DATA_BLOCK DB 15
TITLE =BLOCK DATA FOR TIMER
AUTHOR : Esposito
FAMILY : EGAL_srl
NAME : DB_TD_OP
VERSION : 0.1


  STRUCT
   Axis_press : INT ;	//Value degrees axis rotary press
   Count_tot_R : DINT ;	//Value counter totaly press - read
   Count_par_R : DINT ;	//Value counter partial press - read
   Count_mainte_R : DINT ;	//Value counter maintenance press - read
   Count_par_W : DINT ;	//Value counter partial press - write
   Count_totaly_W : DINT ;	//Value counter totaly - write
   Cam_zero_ON : INT ;	//Value start cam zero - write
   Cam_zero_OFF : INT ;	//Value stop cam zero - write
   Cam_one_ON : INT ;	//Value start cam one - write
   Cam_one_OFF : INT ;	//Value stop cam one - write
   Cam_two_ON : INT ;	//Value start cam two - write
   Cam_two_OFF : INT ;	//Value stop cam two - write
   Cam_three_ON : INT ;	//Value start cam three - write
   Cam_three_OFF : INT ;	//Value stop cam three - write
   Cam_four_ON : INT ;	//Value start cam four - write
   Cam_four_OFF : INT ;	//Value stop cam four - write
   Cam_five_ON : INT ;	//Value start cam five - write
   Cam_five_OFF : INT ;	//Value stop cam five - write
   Cam_six_ON : INT ;	//Value start cam six - write
   Cam_six_OFF : INT ;	//Value stop cam six - write
   Cam_seven_ON : INT ;	//Value start cam seven - write
   Cam_seven_OFF : INT ;	//Value stop cam seven - write
   Cam_eight_ON : INT ;	//Value start cam eight - write
   Cam_eight_OFF : INT ;	//Value stop cam eight - write
   Cam_nine_ON : INT ;	//Value start cam nine - write
   Cam_nine_OFF : INT ;	//Value stop cam nine - write
   Cam_ten_ON : INT ;	//Value start cam ten - write
   Cam_ten_OFF : INT ;	//Value stop cam ten - write
   Cam_eleven_ON : INT ;	//Value start cam eleven - write
   Cam_eleven_OFF : INT ;	//Value stop cam eleven - write
   Cam_twelve_ON : INT ;	//Value start cam twelve - write
   Cam_twelve_OFF : INT ;	//Value stop cam twelve - write
   Cam_thirteen_ON : INT ;	//Value start cam thirteen - write
   Cam_thirteen_OFF : INT ;	//Value stop cam thirteen - write
   Lub_time_pause_R : INT ;	//Value time pause, lubrication pump trabon balancing - read
   Lub_time_job_R : INT ;	//Value time job, lubrication pump trabon balancing - read
   Lub_time_pause_W : INT ;	//Value time pause, lubrication pump trabon balancing - write
   Lub_time_job_W : INT ;	//Value time job, lubrication pump trabon balancing - write
   Overload_POINT1 : REAL ;	//Value point one, pressure overload slide
   Overload_POINT2 : REAL ;	//Value point two, pressure overload slide
   Overload_POINT3 : REAL ;	//Value point three, pressure overload slide
   Overload_POINT4 : REAL ;	//Value point four, pressure overload slide
   Overload_PIW296_R : REAL ;	//Value air pressure, pilotage overload
   Overload_TON288_R : REAL ;	//Value tons overload point one - read
   Overload_TON290_R : REAL ;	//Value tons overload point two - read
   Overload_TON292_R : REAL ;	//Value tons overload point three - read
   Overload_TON294_R : REAL ;	//Value tons overload point four - read
   Ovload_TON_totaly : REAL ;	//Value tons overload totaly slide press - read
   Overload_valve_W : REAL ;	//Value set proportional valve, overload adjustment - write
   Balancing_PIW298_R : REAL ;	//Value air pressure, balancing press - read
   Balancing_value_W : REAL ;	//Value set air pressure, balancing press - write
   Slide_speed_mot_W : REAL ;	//Value set speed slide adjustment press - write
   Slide_value_adju_R : REAL ;	//Value regulation slide adjustment press - read
   Slide_value_adju_W : REAL ;	//Value regulation slide adjustment press - write
   Main_mot_PIW300_R : REAL ;	//Value main motor current press - read
   Main_mot_PIW302_R : REAL ;	//Value main motor speed - read
   Main_mot_PQW306_W : REAL ;	//Value set main motor in stroke - write
   Main_mot_time_OFF_R : INT ;	//Value time main motor, for stop clutch/brake - read
   Main_mot_time_OFF_W : INT ;	//Value time main motor, for stop clutch/brake - write
   Torc_pac_time_OFF_R : INT ;	//Value time cooling torc pac, after stop main motor - read
   Torc_pac_time_OFF_W : INT ;	//Value time cooling torc pac, after stop main motor - write
   Die_safety_prox_R : INT ;	//Value active die safety proximity - read
   Die_safety_prox_W : INT ;	//Value active die safety proximity - write
   Die_coding_R : INT ;	//Value die coding - read
   Die_coding_w : INT ;	//Value die coding - write
   Inlet1_time_PLC_RF : WORD ;	//Value time running, inlet 1 front right upright - read
   Inlet1_time_PLC_WF : INT ;	//Value time running, inlet 1 front right upright - write
   Inlet2_time_PLC_RF : WORD ;	//Value time running, inlet 2 front right upright - read
   Inlet2_time_PLC_WF : INT ;	//Value time running, inlet 2 front right upright - write
   Inlet1_time_PLC_R1R : WORD ;	//Value time running, inlet 1 rear right upright - read
   Inlet1_time_PLC_W1R : INT ;	//Value time running, inlet 1 rear right upright - write
   Inlet2_time_PLC_R2R : WORD ;	//Value time running, inlet 2 rear right upright - read
   Inlet2_time_PLC_W2R : INT ;	//Value time running, inlet 2 rear right upright - write
   Num_prog_Rob1_2_W : INT ;	//Value number program for running, robot 2 - write
   Num_cycle_Rob1_W : INT ;	//Value number cycle for runnig, robot 1  - write
   Num_cycle_Rob2_W : INT ;	//Value number cycle for running, robot 2 - write
   out_PAW304 : REAL ;	//Valore uscita proporz.
   RESERVE : INT ;
   Balan_value : INT ;	//Value from OP_37 for Balancing press
   Elec_cam_ON0 : INT ;	//Electrical cam for cycle 00 - ON
   Elec_cam_OFF0 : INT ;	//Electrical cam for cycle 00 - OFF
   Elec_cam_ON1 : INT ;	//Electrical cam for robot 1 start - ON
   Elec_cam_OFF1 : INT ;	//Electrical cam for robot 1 start - OFF
   Elec_cam_ON2 : INT ;	//Electrical cam for robot 2 start - ON
   Elec_cam_OFF2 : INT ;	//Electrical cam for robot 2 start - OFF
   Elec_cam_ON3 : INT ;	//Electrical cam for safety robot 1 - ON
   Elec_cam_OFF3 : INT ;	//Electrical cam for safety robot 1 - OFF
   Elec_cam_ON4 : INT ;	//Electrical cam for safety robot 2 - ON
   Elec_cam_OFF4 : INT ;	//Electrical cam for safety robot 2 - OFF
   Elec_cam_ON5 : INT ;	//Electrical cam spare - ON
   Elec_cam_OFF5 : INT ;	//Electrical cam spare - OFF
   Elec_cam_ON6 : INT ;	//Electrical cam spare - ON
   Elec_cam_OFF6 : INT ;	//Electrical cam spare - OFF
   Main_mot_min : REAL ;	//Minimal speed main motor press
   Main_mot_max : REAL ;	//Maximal speed main motor press
   Mode_press_cycle : INT ;	//Word for visualize the mode of job press
   Elec_cam_ON7 : INT ;	//Spare cam PLC
   Elec_cam_OFF7 : INT ;	//Spare cam PLC
   Elec_cam_ON8 : INT ;	//Spare cam PLC
   Elec_cam_OFF8 : INT ;	//Spare cam PLC
   Elec_cam_ON9 : INT ;	//Spare cam PLC
   Elec_cam_OFF9 : INT ;	//Spare cam PLC
   Elec_cam_ON10 : INT ;	//Spare cam PLC
   Elec_cam_OFF10 : INT ;	//Spare cam PLC
   Elec_cam_ON11 : INT ;	//Spare cam PLC
   Elec_cam_OFF11 : INT ;	//Spare cam PLC
   Elec_cam_ON12 : INT ;	//Spare cam PLC
   Elec_cam_OFF12 : INT ;	//Spare cam PLC
   Elec_Num_prog : INT ;	//Number cam for load data cam PLC
   Elec_Start_prog : INT ;	//Value cam for load data cam PLC
   Elec_Stop_prog : INT ;	//Value cam for load data cam PLC
   K_parts_counter : INT ;	//Value for conters pices press
  END_STRUCT ;
BEGIN
   Axis_press := 0;
   Count_tot_R := L#250;
   Count_par_R := L#250;
   Count_mainte_R := L#0;
   Count_par_W := L#99999999;
   Count_totaly_W := L#99999999;
   Cam_zero_ON := 0;
   Cam_zero_OFF := 0;
   Cam_one_ON := 0;
   Cam_one_OFF := 0;
   Cam_two_ON := 0;
   Cam_two_OFF := 0;
   Cam_three_ON := 0;
   Cam_three_OFF := 0;
   Cam_four_ON := 0;
   Cam_four_OFF := 0;
   Cam_five_ON := 0;
   Cam_five_OFF := 0;
   Cam_six_ON := 0;
   Cam_six_OFF := 0;
   Cam_seven_ON := 0;
   Cam_seven_OFF := 0;
   Cam_eight_ON := 0;
   Cam_eight_OFF := 0;
   Cam_nine_ON := 0;
   Cam_nine_OFF := 0;
   Cam_ten_ON := 0;
   Cam_ten_OFF := 0;
   Cam_eleven_ON := 0;
   Cam_eleven_OFF := 0;
   Cam_twelve_ON := 0;
   Cam_twelve_OFF := 100;
   Cam_thirteen_ON := 300;
   Cam_thirteen_OFF := 0;
   Lub_time_pause_R := 0;
   Lub_time_job_R := 0;
   Lub_time_pause_W := 999;
   Lub_time_job_W := 15;
   Overload_POINT1 := 0.000000e+000;
   Overload_POINT2 := 0.000000e+000;
   Overload_POINT3 := 0.000000e+000;
   Overload_POINT4 := 0.000000e+000;
   Overload_PIW296_R := 0.000000e+000;
   Overload_TON288_R := 0.000000e+000;
   Overload_TON290_R := 0.000000e+000;
   Overload_TON292_R := 0.000000e+000;
   Overload_TON294_R := 0.000000e+000;
   Ovload_TON_totaly := 0.000000e+000;
   Overload_valve_W := 0.000000e+000;
   Balancing_PIW298_R := 0.000000e+000;
   Balancing_value_W := 0.000000e+000;
   Slide_speed_mot_W := 0.000000e+000;
   Slide_value_adju_R := 0.000000e+000;
   Slide_value_adju_W := 0.000000e+000;
   Main_mot_PIW300_R := 0.000000e+000;
   Main_mot_PIW302_R := 0.000000e+000;
   Main_mot_PQW306_W := 0.000000e+000;
   Main_mot_time_OFF_R := 0;
   Main_mot_time_OFF_W := 0;
   Torc_pac_time_OFF_R := 0;
   Torc_pac_time_OFF_W := 0;
   Die_safety_prox_R := 0;
   Die_safety_prox_W := 0;
   Die_coding_R := 0;
   Die_coding_w := 0;
   Inlet1_time_PLC_RF := W#16#0;
   Inlet1_time_PLC_WF := 0;
   Inlet2_time_PLC_RF := W#16#0;
   Inlet2_time_PLC_WF := 0;
   Inlet1_time_PLC_R1R := W#16#0;
   Inlet1_time_PLC_W1R := 0;
   Inlet2_time_PLC_R2R := W#16#0;
   Inlet2_time_PLC_W2R := 0;
   Num_prog_Rob1_2_W := 1;
   Num_cycle_Rob1_W := 1;
   Num_cycle_Rob2_W := 0;
   out_PAW304 := 0.000000e+000;
   RESERVE := 0;
   Balan_value := 0;
   Elec_cam_ON0 := 0;
   Elec_cam_OFF0 := 0;
   Elec_cam_ON1 := 0;
   Elec_cam_OFF1 := 0;
   Elec_cam_ON2 := 0;
   Elec_cam_OFF2 := 0;
   Elec_cam_ON3 := 0;
   Elec_cam_OFF3 := 0;
   Elec_cam_ON4 := 0;
   Elec_cam_OFF4 := 0;
   Elec_cam_ON5 := 0;
   Elec_cam_OFF5 := 0;
   Elec_cam_ON6 := 0;
   Elec_cam_OFF6 := 0;
   Main_mot_min := 0.000000e+000;
   Main_mot_max := 0.000000e+000;
   Mode_press_cycle := 0;
   Elec_cam_ON7 := 0;
   Elec_cam_OFF7 := 0;
   Elec_cam_ON8 := 0;
   Elec_cam_OFF8 := 0;
   Elec_cam_ON9 := 0;
   Elec_cam_OFF9 := 0;
   Elec_cam_ON10 := 0;
   Elec_cam_OFF10 := 0;
   Elec_cam_ON11 := 0;
   Elec_cam_OFF11 := 0;
   Elec_cam_ON12 := 0;
   Elec_cam_OFF12 := 0;
   Elec_Num_prog := 0;
   Elec_Start_prog := 0;
   Elec_Stop_prog := 0;
   K_parts_counter := 0;
END_DATA_BLOCK

